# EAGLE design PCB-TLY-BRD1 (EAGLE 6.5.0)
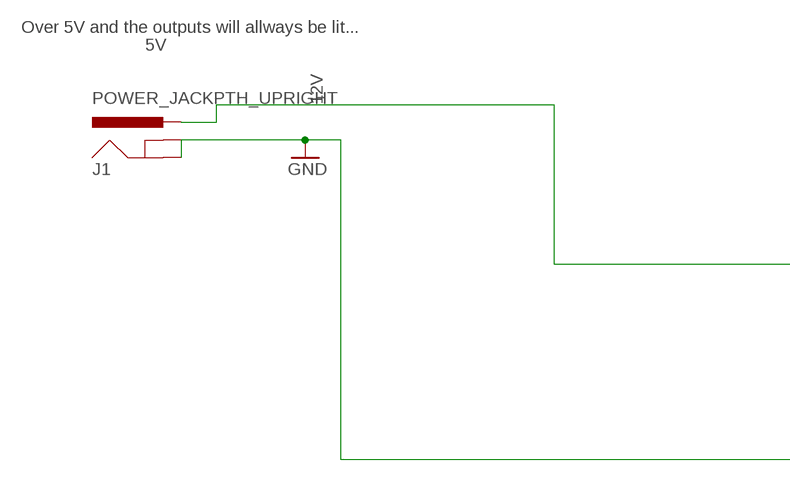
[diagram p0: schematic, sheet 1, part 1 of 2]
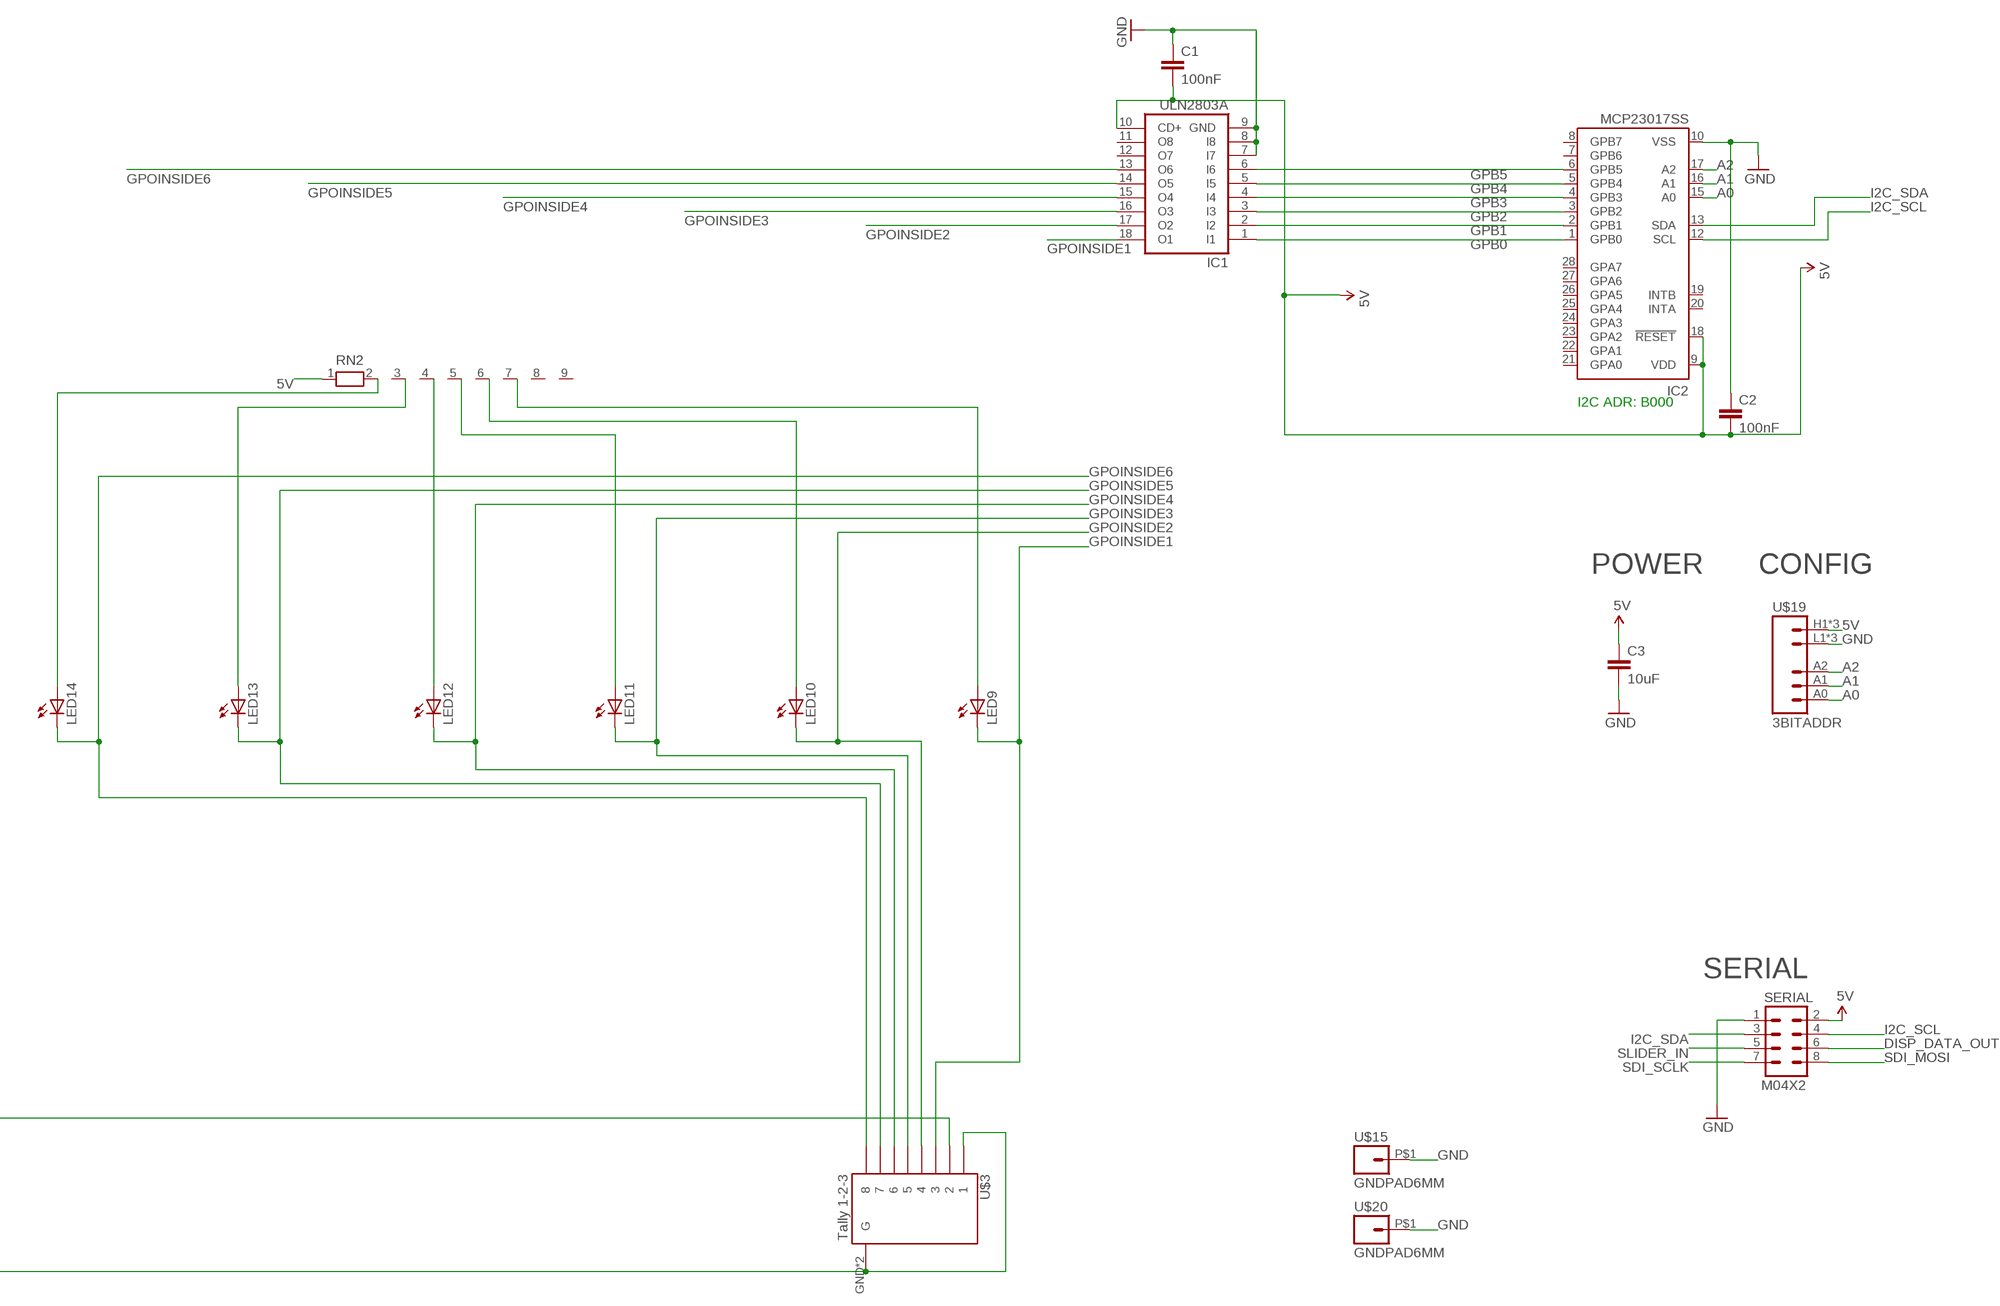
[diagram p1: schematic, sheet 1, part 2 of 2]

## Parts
C1  100nF  CAP0805  [0805]
C2  100nF  CAP0603-CAP  [0603-CAP]
C3  10uF  CAP0805  [0805]
IC1  ULN2803A  ULN2803ASO18W  [SO18W]
IC2  MCP23017SS  [SSOP28]
J1  POWER_JACKPTH_UPRIGHT  [POWER_JACK_PTH_UPRIGHT]
LED9  LED3MM  [LED3MM]
LED10  LED3MM  [LED3MM]
LED11  LED3MM  [LED3MM]
LED12  LED3MM  [LED3MM]
LED13  LED3MM  [LED3MM]
LED14  LED3MM  [LED3MM]
RN2  RN08  [RN-9]
SERIAL  M04X2  [2X4]
U$3  Tally 1-2-3  RJ45-8_GNDUPRIGHT  [RJ45-8_GND_UPRIGHT]
U$15  GNDPAD6MM  [3.2MMPAD6MM]
U$19  3BITADDR  [3BITADDR]
U$20  GNDPAD6MM  [3.2MMPAD6MM]

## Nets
5V [Power]: C1.2 C2.2 C3.1 IC1.10(CD+) IC2.9(VDD) IC2.18(!RESET) RN2.1 SERIAL.2 U$19.H1(VCC) U$19.H2(VCC) U$19.H3(VCC)
12V [Power]: J1.PWR U$3.2
A0: IC2.15(A0) U$19.A0
A1: IC2.16(A1) U$19.A1
A2: IC2.17(A2) U$19.A2
DISP_DATA_OUT: SERIAL.6
GND [Power]: C1.1 C2.1 C3.2 IC1.7(I7) IC1.8(I8) IC1.9(GND) IC2.10(VSS) J1.GND SERIAL.1 U$3.1 U$3.GND1(G) U$3.GND(G) U$15.P$1 U$19.L1(GND) U$19.L2(GND) U$19.L3(GND) U$20.P$1
GPB0: IC1.1(I1) IC2.1(GPB0)
GPB1: IC1.2(I2) IC2.2(GPB1)
GPB2: IC1.3(I3) IC2.3(GPB2)
GPB3: IC1.4(I4) IC2.4(GPB3)
GPB4: IC1.5(I5) IC2.5(GPB4)
GPB5: IC1.6(I6) IC2.6(GPB5)
GPOINSIDE1: IC1.18(O1) LED9.K(C) U$3.3
GPOINSIDE2: IC1.17(O2) LED10.K(C) U$3.4
GPOINSIDE3: IC1.16(O3) LED11.K(C) U$3.5
GPOINSIDE4: IC1.15(O4) LED12.K(C) U$3.6
GPOINSIDE5: IC1.14(O5) LED13.K(C) U$3.7
GPOINSIDE6: IC1.13(O6) LED14.K(C) U$3.8
I2C_SCL: IC2.12(SCL) SERIAL.4
I2C_SDA: IC2.13(SDA) SERIAL.3
N$19: LED14.A RN2.2
N$20: LED13.A RN2.3
N$22: LED12.A RN2.4
N$23: LED11.A RN2.5
N$24: LED10.A RN2.6
N$26: LED9.A RN2.7
SDI_MOSI: SERIAL.8
SDI_SCLK: SERIAL.7
SLIDER_IN: SERIAL.5
Unconnected: IC1.11(O8) IC1.12(O7) IC2.7(GPB6) IC2.8(GPB7) IC2.19(INTB) IC2.20(INTA) IC2.21(GPA0) IC2.22(GPA1) IC2.23(GPA2) IC2.24(GPA3) IC2.25(GPA4) IC2.26(GPA5) IC2.27(GPA6) IC2.28(GPA7) J1.SHUNT(GNDBREAK) RN2.8 RN2.9

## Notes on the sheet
- I2C ADR: B000
- POWER | CONFIG
- Over 5V and the outputs will allways be lit...
- 5V
- SERIAL

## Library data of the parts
C1-C3 = SparkFun:CAP: Capacitor
IC1 = uln-udn:ULN2803A: DRIVER ARRAY
IC2 = microchip:MCP23017: http://ww1.microchip.com/downloads/en/DeviceDoc/21952a.pdf Source: http://ww1.microchip.com/downloads/en/DeviceDoc/21952a.pdf; MF: MICROCHIP; MPN: MCP23017-E/SS; OC_FARNELL: 1467674; OC_NEWARK: 31K2960
J1 = SKAARHOJ:POWER_JACK: RASM712PX Right Angle SMT Mount DC Power Jack, pin size 0.100"(2.5mm), with locating post Switchcraft.com
LED9-LED14 = led:LED: LED
RN2 = SKAARHOJ:RN08: RESISTOR NETWORK; OC_FARNELL: unknown; OC_NEWARK: unknown
SERIAL = SparkFun:M04X2
U$3 = SKAARHOJ:RJ45-8_GND
U$15 U$20 = SKAARHOJ:GNDPAD
U$19 = SKAARHOJ:3BITADDR

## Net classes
0 default: width 0.203 mm, drill 0.406 mm, clearance 0.203 mm
1 Power: width 0.406 mm, drill 0.61 mm, clearance 0.203 mm
2 RELAY LINES: width 0.305 mm, clearance 0.254 mm
3 INput lines: clearance 0.254 mm

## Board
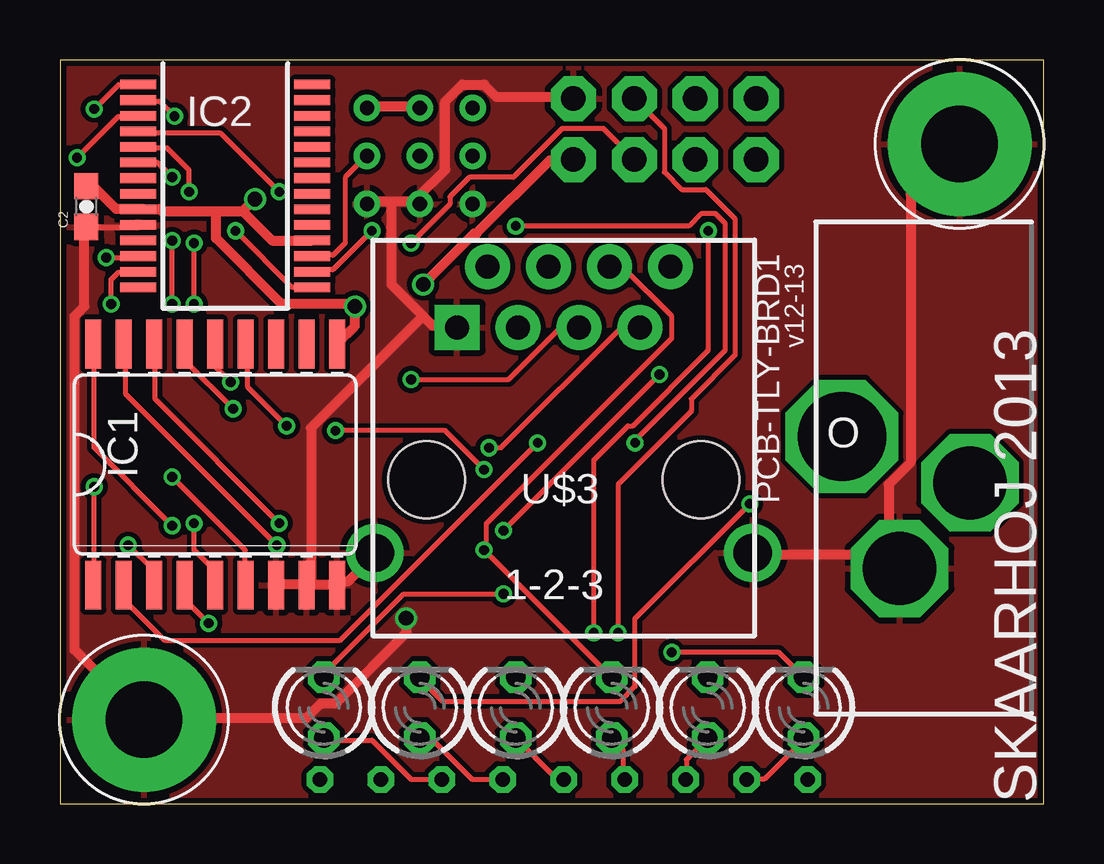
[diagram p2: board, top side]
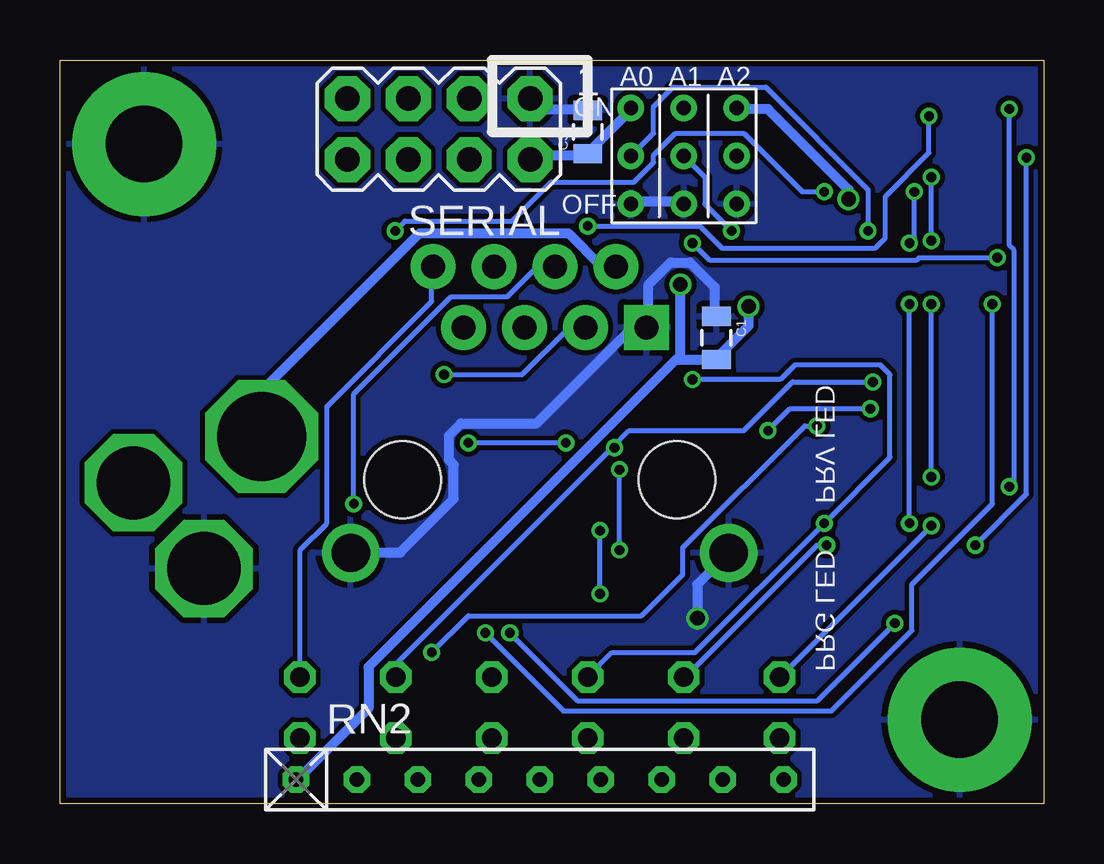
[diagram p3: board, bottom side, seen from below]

Size 41 x 31 mm. Coordinates in mm from the lower left corner, seen from the top.
Outline: 41,0 41,31 0,31 0,0 41,0
Copper layers (1*16): Top 0.035mm / dielectric 1.5mm / Bottom 0.035mm
Design rules "Fusion_eagle_rule_v1.1": minimum track width 6mil, minimum drill 12mil, track to track 6mil, track to pad 6mil, pad to pad 6mil, via to via 6mil, smd to smd 0mil, copper to edge 10mil, drill to drill 10mil, minimum pad ring 10mil, minimum via ring 6mil, stop-mask expansion 2mil, vias tented up to drill 100mil, thermal gap 10mil
bKeepout: area 0,0 to 10,10; area 140,0 to 150,10

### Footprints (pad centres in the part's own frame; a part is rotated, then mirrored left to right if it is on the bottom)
0805 = smd 0.8 x 1.2: 1 -0.9,0; 2 0.9,0
0603-CAP = smd 1.1 x 1: 1 -0.85,0; 2 0.85,0
SO18W = smd 0.66 x 2.032: 1 -5.08,-5.029; 2 -3.81,-5.029; 3 -2.54,-5.029; 4 -1.27,-5.029; 5 0,-5.029; 6 1.27,-5.029; 7 2.54,-5.029; 8 3.81,-5.029; 9 5.08,-5.029; 10 5.08,5.029; 11 3.81,5.029; 12 2.54,5.029; 13 1.27,5.029; 14 0,5.029; 15 -1.27,5.029; 16 -2.54,5.029; 17 -3.81,5.029; 18 -5.08,5.029
SSOP28 = smd 0.4 x 1.5: 1 -4.225,-3.625; 2 -3.575,-3.625; 3 -2.925,-3.625; 4 -2.275,-3.625; 5 -1.625,-3.625; 6 -0.975,-3.625; 7 -0.325,-3.625; 8 0.325,-3.625; 9 0.975,-3.625; 10 1.625,-3.625; 11 2.275,-3.625; 12 2.925,-3.625; 13 3.575,-3.625; 14 4.225,-3.625; 15 4.225,3.625; 16 3.575,3.625; 17 2.925,3.625; 18 2.275,3.625; 19 1.625,3.625; 20 0.975,3.625; 21 0.325,3.625; 22 -0.325,3.625; 23 -0.975,3.625; 24 -1.625,3.625; 25 -2.275,3.625; 26 -2.925,3.625; 27 -3.575,3.625; 28 -4.225,3.625
POWER_JACK_PTH_UPRIGHT = drill 3.048 octagon: GND -1,-4.2; SHUNT 1.935,-0.63 | drill 3.7 octagon: PWR -3.4,1.3
LED3MM = drill 0.813 octagon: A -1.27,0; K 1.27,0
RN-9 = drill 0.6 octagon: 1 -10.16,0; 2 -7.62,0; 3 -5.08,0; 4 -2.54,0; 5 0,0; 6 2.54,0; 7 5.08,0; 8 7.62,0; 9 10.16,0
2X4 = drill 1.016 pad 1.88 octagon: 1 -3.81,-1.27; 2 -3.81,1.27; 3 -1.27,-1.27; 4 -1.27,1.27; 5 1.27,-1.27; 6 1.27,1.27; 7 3.81,-1.27; 8 3.81,1.27
RJ45-8_GND_UPRIGHT = drill 1 pad 1.88 square: 1 -4.445,6.35 | drill 1 pad 1.88: 2 -3.175,8.89; 3 -1.905,6.35; 4 -0.635,8.89; 5 0.635,6.35; 6 1.905,8.89; 7 3.175,6.35; 8 4.445,8.89 | drill 1.6: GND -7.88,-3.05; GND1 7.88,-3.05 | hole 3.2: -5.715,0; 5.715,0
3.2MMPAD6MM = drill 3.2 pad 6: P$1 0,0
3BITADDR = drill 0.6: A0 -2.2,0; A1 0,0; A2 2.2,0; H1 -2.2,2; H2 0,2; H3 2.2,2; L1 -2.2,-2; L2 0,-2; L3 2.2,-2

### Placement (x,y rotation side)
C1  13.63,19.41 270 bottom
C2  1.1,24.89 90 top
C3  19,28 90 bottom
IC1  6.47,14.13 0 top
IC2  6.89,25.75 270 top
J1  36,14 0 top
LED9  11,4 90 top
LED10  15,4 90 top
LED11  19,4 90 top
LED12  23,4 90 top
LED13  27,4 90 top
LED14  31,4 90 top
RN2  21,1 0 bottom
SERIAL  25.21,28.12 180 bottom
U$3  21,13.5 0 top
U$15  3.5,3.5 0 top
U$19  15,27 0 bottom
U$20  37.5,27.5 0 top

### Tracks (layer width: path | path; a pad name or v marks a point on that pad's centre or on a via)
5V  (via drill 0.61)
  Top 0.406: U$19.H3 12.8,29.06 14.94,29.06 U$19.H2 | C2.2 1.12,25.7 1.42,25.7 2.34,24.79 3.25,24.79 IC2.9 3.45,24.79 4.17,24.79 4.27,24.69 6.5,24.69 | 7.62,24.69 8.84,23.47 10.46,23.47 IC2.18 | 6.5,24.69 7.62,24.69 | 7.62,24.69 v8.13,25.2 | IC1.10 11.58,19.2 12.29,19.91 v12.29,20.73 12.19,20.83 9.25,20.83 6.5,23.57 6.5,24.69 | v15.14,21.64 17.27,23.77 17.37,23.77 20.42,26.82 21.34,26.82 SERIAL.2
  Bottom 0.406: v8.13,25.2 8.13,25.6 11.48,28.96 12.7,28.96 U$19.H3 | U$19.H1 17.17,28.96 19,27.13 C3.1 19.2,27.03 21.23,27.03 21.34,26.92 SERIAL.2 | v12.29,20.73 12.29,19.91 13.61,18.59 C1.2 13.82,18.49 15.14,18.49 | 15.14,18.49 15.34,18.49 28.14,5.69 28.14,3.96 31.09,1.02 RN2.1 | 15.14,18.49 v15.14,21.64
12V
  Bottom 0.406: U$3.2 17.88,22.45 18.49,22.45 19.81,23.77 26.01,23.77 32.51,17.27 32.51,15.34 J1.PWR
A0  (via drill 0.41)
  Top 0.203: v7.32,23.88 9.65,21.54 10.46,21.54 IC2.15
  Bottom 0.203: v7.32,23.88 7.32,25.6 11.58,29.87 15.44,29.87 16.26,29.06 16.26,27.94 17.17,27.03 U$19.A0
A1  (via drill 0.41)
  Top 0.203: v13.01,23.88 11.38,22.25 10.57,22.25 IC2.16
  Bottom 0.203: v13.01,23.88 14.12,24.99 14.12,26.11 14.94,26.92 U$19.A1
A2
  Top 0.203: IC2.17 10.57,22.86 11.38,22.86 11.89,23.37 11.89,26.11 12.7,26.92 U$19.A2
GND  (via drill 0.61)
  Top 0.254: C2.1 3.27,24.04 IC2.10
  Top 0.406: C2.1 1.02,23.98 1.02,20.73 0.61,20.32 0.61,6.4 3.45,3.56 U$15.P$1 3.66,3.56 10.26,3.56 10.87,4.17 11.48,4.17 14.43,7.11 v14.43,7.72 | IC1.7 9.04,9.14 10.26,9.14 IC1.8 | IC1.8 10.46,9.14 11.48,9.14 IC1.9 11.68,9.25 11.99,9.25 13.11,10.36 U$3.GND | 13.82,25.09 14.94,25.09 U$19.L2 14.94,25.3 16.05,26.42 16.05,29.26 16.76,29.97 17.68,29.97 18.19,29.46 21.34,29.46 SERIAL.1 | 13.82,25.09 12.8,25.09 U$19.L3 | 13.82,25.09 13.82,21.64 15.14,20.32 | 15.14,20.32 15.54,19.91 16.46,19.91 U$3.1 | 15.14,20.32 10.46,15.65 10.46,9.35 IC1.8 | U$3.GND1 28.96,10.36 34.44,10.36 34.95,9.86 J1.GND 34.54,10.46 34.54,13.31 35.46,14.22 35.46,25.4 37.49,27.43 U$20.P$1
  Bottom 0.406: C3.2 19.1,28.96 20.93,28.96 21.34,29.36 SERIAL.1 | U$19.L1 17.17,25.09 15.04,25.09 U$19.L2 | C1.1 13.72,20.32 13.72,21.54 14.73,22.55 15.54,22.55 16.46,21.64 16.46,19.91 U$3.1 16.76,19.81 17.17,19.81 21.13,15.85 24.28,15.85 24.79,15.34 24.79,14.33 24.59,14.12 24.59,12.7 26.82,10.46 28.85,10.46 U$3.GND1 | v14.43,7.72 14.43,9.14 13.21,10.36 U$3.GND
  pour Top: 0,0 41,0 41,31 0,31
  pour Bottom: 0,0 41,0 41,31 0,31
GPB0  (via drill 0.41)
  Top 0.203: v1.42,28.96 2.44,29.97 IC2.1 | v1.42,13.21 1.42,9.14 IC1.1
  Bottom 0.203: v1.42,28.96 1.42,23.27 1.22,23.06 1.22,13.41 v1.42,13.21
GPB1  (via drill 0.41)
  Top 0.203: v4.78,28.65 4.17,29.26 3.35,29.26 IC2.2 | v19,24.08 26.21,24.08 26.72,24.59 27.33,24.59 27.74,24.18 27.74,18.9 23.98,15.14 v23.98,15.04 | v19.91,15.04 11.68,6.81 4.37,6.81 2.74,8.43 2.74,9.04 IC1.2
  Bottom 0.203: v4.78,28.65 4.78,27.13 6.6,25.3 6.6,23.57 7.01,23.16 13.41,23.16 14.33,24.08 v19,24.08 | v19.91,15.04 v23.98,15.04
GPB2  (via drill 0.41)
  Top 0.203: v0.71,26.92 2.44,28.65 3.25,28.65 IC2.3 | v2.85,10.77 3.86,9.75 3.86,9.14 IC1.3
  Bottom 0.203: v0.71,26.92 0.71,12.9 v2.85,10.77
GPB3  (via drill 0.41)
  Top 0.203: v9.14,25.5 6.71,27.94 3.35,27.94 IC2.4 | v27.03,23.88 27.03,18.9 23.88,15.75 23.67,15.75 22.25,14.33 v22.25,7.11 | v6.2,7.52 5.28,8.43 5.28,9.04 IC1.4
  Bottom 0.203: v9.14,25.5 10.06,25.5 12.5,27.94 15.34,27.94 16.26,27.03 16.26,26.72 17.07,25.91 20.52,25.91 22.15,24.28 26.62,24.28 v27.03,23.88 | v22.25,7.11 19.41,4.27 9.45,4.27 v6.2,7.52
GPB4  (via drill 0.41)
  Top 0.203: v5.38,25.5 5.38,26.42 4.47,27.33 3.35,27.33 IC2.5 | v5.59,20.83 v5.59,23.37 | v5.59,11.68 5.59,10.57 6.4,9.75 6.4,9.14 IC1.5
  Bottom 0.203: v5.38,25.5 5.38,23.57 v5.59,23.37 | v5.59,11.68 v5.59,20.83
GPB5  (via drill 0.41)
  Top 0.203: v4.67,26.11 4.06,26.72 3.35,26.72 IC2.6 | v4.67,20.83 v4.67,23.47 | v4.67,13.61 7.72,10.57 7.72,9.14 IC1.6
  Bottom 0.203: v4.67,23.47 v4.67,26.11 | v4.67,13.61 v4.67,20.83
GPOINSIDE1  (via drill 0.41)
  Top 0.203: v4.67,11.58 1.42,14.83 1.42,19.1 IC1.18 | v18.49,11.38 v24.99,17.88 | v18.49,8.74 14.33,8.74 11.07,5.49 11.07,5.28 LED9.K
  Bottom 0.203: v4.67,11.58 10.97,5.28 LED9.K | v24.99,17.88 21.74,17.88 19.81,19.81 19.1,19.81 U$3.3 | v18.49,8.74 v18.49,11.38
GPOINSIDE2  (via drill 0.41)
  Top 0.203: v9.04,10.77 2.74,17.07 2.74,19.1 IC1.17 | v28.75,12.5 23.98,7.72 23.98,4.88 23.37,4.27 15.95,4.27 15.04,5.18 LED10.K
  Bottom 0.203: v9.04,10.77 9.45,10.77 14.94,5.28 LED10.K | v28.75,12.5 28.75,17.07 24.69,21.13 22.35,21.13 21.13,22.35 20.42,22.35 U$3.4
GPOINSIDE3  (via drill 0.41)
  Top 0.203: v9.14,11.68 3.96,16.87 3.96,19.1 IC1.16 | v14.63,17.68 18.69,17.68 20.83,19.81 21.54,19.81 U$3.5
  Bottom 0.203: LED11.K 19,5.28 17.98,6.3 14.53,6.3 v9.14,11.68 6.4,14.43 6.4,17.88 6.81,18.29 10.36,18.29 10.97,17.68 v14.63,17.68
GPOINSIDE4  (via drill 0.41)
  Top 0.203: v7.21,16.46 5.28,18.39 5.28,19.1 IC1.15 | v11.48,15.54 16.05,15.54 v17.68,13.92 | LED12.K 22.96,5.28 v17.68,10.57 17.78,10.57 17.78,11.68 25.5,19.41 25.5,20.32 23.47,22.35 22.96,22.35 U$3.6
  Bottom 0.203: v7.21,16.46 10.57,16.46 v11.48,15.54 | v17.68,10.57 v17.68,13.92
GPOINSIDE5  (via drill 0.41)
  Top 0.203: v7.11,17.58 6.5,18.19 6.5,19.1 IC1.14 | v17.88,14.83 18.39,14.83 23.37,19.81 24.08,19.81 U$3.7
  Bottom 0.203: v7.11,17.58 10.46,17.58 12.5,15.54 17.27,15.54 17.93,14.88 | 17.93,14.88 26.92,5.89 26.92,5.28 LED13.K | v17.88,14.83 17.93,14.88
GPOINSIDE6  (via drill 0.41)
  Top 0.203: v9.45,15.75 7.82,17.37 7.82,19.1 IC1.13 | v25.5,6.3 29.97,6.3 30.99,5.28 LED14.K
  Bottom 0.203: v9.45,15.75 9.96,15.75 15.04,10.67 15.04,9.55 16.76,7.82 23.98,7.82 v25.5,6.3 | U$3.8 25.5,22.35 25.5,20.93 29.87,16.56 29.87,11.68 30.99,10.57 30.99,5.28 LED14.K
I2C_SCL  (via drill 0.41)
  Top 0.203: v1.93,22.76 3.25,22.76 IC2.12 | v14.63,23.37 16.26,24.99 16.26,25.3 17.07,26.11 18.9,26.11 20.93,28.14 22.66,28.14 23.88,26.92 SERIAL.4
  Bottom 0.203: v1.93,22.76 5.18,22.76 5.28,22.66 13.92,22.66 v14.63,23.37
I2C_SDA  (via drill 0.41)
  Top 0.203: v2.13,20.83 2.13,21.84 2.44,22.15 3.25,22.15 IC2.13 | v23.27,7.11 23.27,13.31 26.31,16.36 26.31,16.87 28.14,18.69 28.14,24.38 26.92,25.6 25.91,25.6 25.2,26.31 25.2,28.14 23.98,29.36 SERIAL.3
  Bottom 0.203: v2.13,20.83 2.13,12.5 5.49,9.14 5.49,7.21 8.84,3.86 20.02,3.86 v23.27,7.11
N$19
  Top 0.203: RN2.2 28.65,1.02 29.36,1.02 30.99,2.64 LED14.A
N$20
  Top 0.203: RN2.3 26.11,1.02 26.11,1.83 26.92,2.64 LED13.A
N$22
  Top 0.203: RN2.4 23.47,1.02 23.47,2.23 23.06,2.64 LED12.A
N$23
  Top 0.203: RN2.5 20.93,1.02 20.73,1.02 19.1,2.64 LED11.A
N$24
  Top 0.203: RN2.6 18.39,1.02 17.17,1.02 15.54,2.64 15.04,2.64 LED10.A
N$26
  Top 0.203: RN2.7 15.85,1.02 14.63,1.02 13.01,2.64 11.07,2.64 LED9.A

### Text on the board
_tsilk: v12-13 | O | PCB-TLY-BRD1 | 1-2-3 | SKAARHOJ 2013
_bsilk: 1 | PRV LED | PRG LED

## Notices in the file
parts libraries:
SparkFun: Licensing: CC v3.0 Share-Alike You are welcome to use this library for commercial purposes.
